(* Logix 5000 Rung export; software revision 33.00 *)

TYPE Banner_IOL_Device_SubIndex :
STRUCT
   Sub : DINT[34];
END_STRUCT
END_TYPE

TYPE Banner_IOL_QM30VT3_Device :
STRUCT
   Initial_Global_Read : BOOL;
   Command : SINT;
   Data : Banner_IOL_QM30VT3_Device_Index;
   Reset : BOOL;
END_STRUCT
END_TYPE

TYPE Banner_IOL_QM30VT3_Device_Index :
STRUCT
   Index : Banner_IOL_Device_SubIndex[19];
   Metric_Config : Banner_IOL_QM30VT3_Metric_Config;
END_STRUCT
END_TYPE

TYPE Banner_IOL_QM30VT3_Metric_Config :
STRUCT
   Metric_1 : Banner_IOL_QM30VT3_Metric_Data;
   Metric_2 : Banner_IOL_QM30VT3_Metric_Data;
   Metric_3 : Banner_IOL_QM30VT3_Metric_Data;
   Metric_4 : Banner_IOL_QM30VT3_Metric_Data;
   Metric_5 : Banner_IOL_QM30VT3_Metric_Data;
   Metric_6 : Banner_IOL_QM30VT3_Metric_Data;
   Metric_7 : Banner_IOL_QM30VT3_Metric_Data;
   Num_of_Threshold_Samples : DINT;
END_STRUCT
END_TYPE

TYPE Banner_IOL_QM30VT3_Metric_Data :
STRUCT
   Metric : DINT;   // See IODD file for all options.
   Warning_Threshold : REAL;
   Alarm_Treshold : REAL;
END_STRUCT
END_TYPE

TYPE Banner_IOL_Rules :
STRUCT
   Byte_Pos : SINT;   // Byte Position to read from or write data to.
   Multi : SINT;   // Determines if a multiple byte length index is being accessed. Use 2 for 2 bytes length, 3 for 3 byte length, etc..
   Sub_Index : SINT;
   Signed : SINT;   // 0=Unsigned, 1=Signed
END_STRUCT
END_TYPE

TYPE Banner_IOL_Rules_Array :
STRUCT
   Length : DINT;
   Settings : Banner_IOL_Rules_SettingsArray[32];
END_STRUCT
END_TYPE

TYPE Banner_IOL_Rules_SettingsArray :
STRUCT
   Index : DINT;
   Num_Op : INT;   // Number of Operations to read/write Index.
   Total_Bytes : INT;
   RW : SINT;   // 0 = Read Only, 1 = Write Only, 2 = Read or Write
   Rules : Banner_IOL_Rules[34];   // Sub Index Position in IODD.
END_STRUCT
END_TYPE

VAR_GLOBAL   (* controller tags *)
   QM30VT3_IOLM1_01 : Banner_IOL_QM30VT3_Device;
        .DATA.INDEX[2]   // Direct Parameters 1 (ro)
        .DATA.INDEX[2].SUB[1]   // Reserved
        .DATA.INDEX[2].SUB[2]   // Master Cycle Time
        .DATA.INDEX[2].SUB[3]   // Min Cycle Time
        .DATA.INDEX[2].SUB[4]   // M Sequence Capability
        .DATA.INDEX[2].SUB[5]   // IO-Link Version ID
        .DATA.INDEX[2].SUB[6]   // Process Data Input Length
        .DATA.INDEX[2].SUB[7]   // Process Data Output Length
        .DATA.INDEX[2].SUB[8]   // Vendor ID
        .DATA.INDEX[2].SUB[9]   // Device ID
        .DATA.INDEX[3]   // Standard Command (wo)
        .DATA.INDEX[3].SUB[1]   // Standard Command: 126=Locator Start, 127=Locator Stop, 129=Application Reset, 164=Reset All Metrics
        .DATA.INDEX[4]   // Serial Number (ro)
        .DATA.INDEX[4].SUB[1]   // SN1
        .DATA.INDEX[4].SUB[2]   // SN2
        .DATA.INDEX[4].SUB[3]   // SN3
        .DATA.INDEX[4].SUB[4]   // SN4
        .DATA.INDEX[4].SUB[5]   // SN5
        .DATA.INDEX[4].SUB[6]   // SN6
        .DATA.INDEX[4].SUB[7]   // SN7
        .DATA.INDEX[4].SUB[8]   // SN8
        .DATA.INDEX[4].SUB[9]   // SN9
        .DATA.INDEX[4].SUB[10]   // SN10
        .DATA.INDEX[4].SUB[11]   // SN11
        .DATA.INDEX[4].SUB[12]   // SN12
        .DATA.INDEX[4].SUB[13]   // SN13
        .DATA.INDEX[4].SUB[14]   // SN14
        .DATA.INDEX[4].SUB[15]   // SN15
        .DATA.INDEX[4].SUB[16]   // SN16
        .DATA.INDEX[5]   // All Time Run Time (ro)
        .DATA.INDEX[5].SUB[1]   // All Time Run Time
        .DATA.INDEX[6]   // Resettable Run Time
        .DATA.INDEX[6].SUB[1]   // Resettable Run Time
        .DATA.INDEX[7]   // Process Data Mode
        .DATA.INDEX[7].SUB[1]   // Process Data Mode: 0=FP Imperial, 1=SSP Imperial, 2=FP Metric, 3=SSP Metric, 4=FP User Define, 5=SSP User Define
        .DATA.INDEX[8]   // Output Configuration
        .DATA.INDEX[8].SUB[1]   // Wire Mode: 0=BannerBus, 1=Discrete Output
        .DATA.INDEX[9]   // Reserved
        .DATA.INDEX[9].SUB[1]   // Metric 1
        .DATA.INDEX[9].SUB[2]   // Metric 1 Warning Threshold
        .DATA.INDEX[9].SUB[3]   // Metric 1 Alarm Threshold
        .DATA.INDEX[9].SUB[4]   // Metric 2
        .DATA.INDEX[9].SUB[5]   // Metric 2 Warning Threshold
        .DATA.INDEX[9].SUB[6]   // Metric 2 Alarm Threshold
        .DATA.INDEX[9].SUB[7]   // Metric 3
        .DATA.INDEX[9].SUB[8]   // Metric 3 Warning Threshold
        .DATA.INDEX[9].SUB[9]   // Metric 3 Alarm Threshold
        .DATA.INDEX[9].SUB[10]   // Metric 4
        .DATA.INDEX[9].SUB[11]   // Metric 4 Warning Threshold
        .DATA.INDEX[9].SUB[12]   // Metric Alarm Threshold
        .DATA.INDEX[9].SUB[13]   // Metric 5
        .DATA.INDEX[9].SUB[14]   // Metric 5 Warning Threshold
        .DATA.INDEX[9].SUB[15]   // Metric 5 Alarm Threshold
        .DATA.INDEX[9].SUB[16]   // Metric 6
        .DATA.INDEX[9].SUB[17]   // Metric 6 Warning Threshold
        .DATA.INDEX[9].SUB[18]   // Metric 6 Alarm Threshold
        .DATA.INDEX[9].SUB[19]   // Metric 7 Alarm Threshold
        .DATA.INDEX[9].SUB[20]   // Metric 7 Warning Threshold
        .DATA.INDEX[9].SUB[21]   // Metric 7 Alarm Threshold
        .DATA.INDEX[9].SUB[22]   // Number of Threshold Samples
        .DATA.INDEX[10]   // Status (ro)
        .DATA.INDEX[10].SUB[1]   // Vibe IQ Status: 0=IDLE, 1=Start, 2=Samples Acquiring, 3=Processing, 4=Active
        .DATA.INDEX[10].SUB[2]   // Baseline Sample Left
        .DATA.INDEX[11]   // Vibe IQ Sampling
        .DATA.INDEX[11].SUB[1]   // FMAx Settings: 1=Fmax 5300 Hz, 2=Fmax 2650 Hz, 3=Fmax 1300 Hz, 4=Fmax 650 Hz, 5=Fmax 325 Hz
        .DATA.INDEX[12]   // Baseline Configuration
        .DATA.INDEX[12].SUB[1]   // Start Baseline: 0=Idle, 1=Trigger Baseline, 2=Baseline Abord/Reset
        .DATA.INDEX[12].SUB[2]   // Velocity Threshold Compare: 0=Velocity Threshold or with Axis, 1=Velocity Threshold and with Axis
        .DATA.INDEX[12].SUB[3]   // Accel Component for Threshold: 0 to 65535
        .DATA.INDEX[12].SUB[4]   // Accel Velocity or and Threshold Exceed for Baseline: 0 to 65535
        .DATA.INDEX[12].SUB[5]   // Number of Samples for Baseline: 0 to 65535
        .DATA.INDEX[12].SUB[6]   // Sample Rate in seconds for Baseline: 0 to 65535
        .DATA.INDEX[12].SUB[7]   // Number of Samples for Acute: 0 to 65535
        .DATA.INDEX[12].SUB[8]   // Number of Samples for Chronic: 0 to 65535
        .DATA.INDEX[12].SUB[9]   // Imperial or Metric Selection: 0=Imperial, 1=Metric
        .DATA.INDEX[13]   // Baseline Threshold Configuration
        .DATA.INDEX[13].SUB[1]   // X RMS Velocity Threshold for Baseline: 0 to 65535
        .DATA.INDEX[13].SUB[2]   // Y RMS Velocity Threshold for Baseline: 0 to 65535
        .DATA.INDEX[13].SUB[3]   // Z RMS Velocity Threshold for Baseline: 0 to 65535
        .DATA.INDEX[13].SUB[4]   // X RMS HP Accel Threshold for Baseline: 0 to 65535
        .DATA.INDEX[13].SUB[5]   // Y RMS HP Accel Threshold for Baseline: 0 to 65535
        .DATA.INDEX[13].SUB[6]   // Z RMS HP Accel Threshold for Baseline: 0 to 65535
        .DATA.INDEX[14]   // Baseline Avg Configuration
        .DATA.INDEX[14].SUB[1]   // X RMS Velocity Vib Baseline: 0 to 65535
        .DATA.INDEX[14].SUB[2]   // Y RMS Velocity Vib Baseline: 0 to 65535
        .DATA.INDEX[14].SUB[3]   // Z RMS Velocity Vib Baseline: 0 to 65535
        .DATA.INDEX[14].SUB[4]   // X RMS HP Accel Vibration Baseline: 0 to 65535
        .DATA.INDEX[14].SUB[5]   // Y RMS HP Accel Vibration Baseline: 0 to 65535
        .DATA.INDEX[14].SUB[6]   // Z RMS HP Accel Vibration Baseline: 0 to 65535
        .DATA.INDEX[15]   // Baseline Warning Threshold Configuration
        .DATA.INDEX[15].SUB[1]   // X RMS Velocity Warning Threshold: 0 to 65535
        .DATA.INDEX[15].SUB[2]   // Y RMS Velocity Warning Threshold: 0 to 65535
        .DATA.INDEX[15].SUB[3]   // Z RMS Velocity Warning Threshold: 0 to 65535
        .DATA.INDEX[15].SUB[4]   // X RMS HP Accel Warning Threshold: 0 to 65535
        .DATA.INDEX[15].SUB[5]   // Y RMS HP Accel Warning Threshold: 0 to 65535
        .DATA.INDEX[15].SUB[6]   // Z RMS HP Accel Warning Threshold: 0 to 65535
        .DATA.INDEX[16]   // Baseline Alarm Threshold Configuration
        .DATA.INDEX[16].SUB[1]   // X RMS Velocity Alarm Threshold: 0 to 65535
        .DATA.INDEX[16].SUB[2]   // Y RMS Velocity Alarm Threshold: 0 to 65535
        .DATA.INDEX[16].SUB[3]   // Z RMS Velocity Alarm Threshold: 0 to 65535
        .DATA.INDEX[16].SUB[4]   // X RMS HP Accel Alarm Threshold: 0 to 65535
        .DATA.INDEX[16].SUB[5]   // Y RMS HP Accel Alarm Threshold: 0 to 65535
        .DATA.INDEX[16].SUB[6]   // Z RMS HP Accel Alarm Threshold: 0 to 65535
        .DATA.INDEX[17]   // Baseline Temp Alarm Warning Threshold
        .DATA.INDEX[17].SUB[1]   // Temp Warning Treshold Value: 0 to 65535
        .DATA.INDEX[17].SUB[2]   // Temp Alarm Threshold Value: 0 to 65535
        .DATA.METRIC_CONFIG   // Index 9
   QM30VT3_Rules : Banner_IOL_Rules_Array;
        .SETTINGS[2]   // Direct Parameters 1
        .SETTINGS[2].RULES[0]   // Reserved
        .SETTINGS[2].RULES[1]   // Master Cycle Time
        .SETTINGS[2].RULES[2]   // Min Cycle Time
        .SETTINGS[2].RULES[3]   // M-Sequence Capability
        .SETTINGS[2].RULES[4]   // IO-Link ID
        .SETTINGS[2].RULES[5]   // Process Data Input Length
        .SETTINGS[2].RULES[6]   // Process Data Output Length
        .SETTINGS[2].RULES[7]   // Vendor ID
        .SETTINGS[2].RULES[8]   // Device ID
        .SETTINGS[3]   // Standard Command
        .SETTINGS[3].RULES[0]   // Standard Command
        .SETTINGS[4]   // Serial Number
        .SETTINGS[4].RULES[0]   // SN1
        .SETTINGS[4].RULES[1]   // SN2
        .SETTINGS[4].RULES[2]   // SN3
        .SETTINGS[4].RULES[3]   // SN4
        .SETTINGS[4].RULES[4]   // SN5
        .SETTINGS[4].RULES[5]   // SN6
        .SETTINGS[4].RULES[6]   // SN7
        .SETTINGS[4].RULES[7]   // SN8
        .SETTINGS[4].RULES[8]   // SN9
        .SETTINGS[4].RULES[9]   // SN10
        .SETTINGS[4].RULES[10]   // SN11
        .SETTINGS[4].RULES[11]   // SN12
        .SETTINGS[4].RULES[12]   // SN13
        .SETTINGS[4].RULES[13]   // SN14
        .SETTINGS[4].RULES[14]   // SN15
        .SETTINGS[4].RULES[15]   // SN16
        .SETTINGS[5]   // All Time Run Time
        .SETTINGS[5].RULES[0]   // All Time Run Time
        .SETTINGS[6]   // Resettable Run Time
        .SETTINGS[6].RULES[0]   // Resettable Run Time
        .SETTINGS[7]   // Process Data Mode
        .SETTINGS[7].RULES[0]   // Process Data Mode
        .SETTINGS[8]   // Output Configuration
        .SETTINGS[8].RULES[0]   // Output Configuration
        .SETTINGS[9]   // Metric Configuration
        .SETTINGS[9].RULES[0]   // Metric 1
        .SETTINGS[9].RULES[1]   // Metric 1 Warning Threshold
        .SETTINGS[9].RULES[2]   // Metric 1 Alarm Threshold
        .SETTINGS[9].RULES[3]   // Metric 2
        .SETTINGS[9].RULES[4]   // Metric 2 Warning Threshold
        .SETTINGS[9].RULES[5]   // Metric 2 Alarm Threshold
        .SETTINGS[9].RULES[6]   // Metric 3
        .SETTINGS[9].RULES[7]   // Metric 3 Warning Threshold
        .SETTINGS[9].RULES[8]   // Metric 3 Alarm Threshold
        .SETTINGS[9].RULES[9]   // Metric 4
        .SETTINGS[9].RULES[10]   // Metric 4 Warning Threshold
        .SETTINGS[9].RULES[11]   // Metric 4 Alarm Threshold
        .SETTINGS[9].RULES[12]   // Metric 5
        .SETTINGS[9].RULES[13]   // Metric 5 Warning Threshold
        .SETTINGS[9].RULES[14]   // Metric 5 Alarm Threshold
        .SETTINGS[9].RULES[15]   // Metric 6
        .SETTINGS[9].RULES[16]   // Metric 6 Warning Threshold
        .SETTINGS[9].RULES[17]   // Metric 6 Alarm Threshold
        .SETTINGS[9].RULES[18]   // Metric 7
        .SETTINGS[9].RULES[19]   // Metric 7 Warning Threshold
        .SETTINGS[9].RULES[20]   // Metric 7 Alarm Threshold
        .SETTINGS[9].RULES[21]   // Number of Threshold Samples
        .SETTINGS[10]   // Status
        .SETTINGS[10].RULES[0]   // Vibe IQ Status
        .SETTINGS[10].RULES[1]   // Baseline Sample Left
        .SETTINGS[11]   // Vibe IQ Sampling
        .SETTINGS[11].RULES[0]   // FMax Settings
        .SETTINGS[12]   // Baseline Configuration
        .SETTINGS[12].RULES[0]   // Start Baseline
        .SETTINGS[12].RULES[1]   // Velocity Threshold Compare
        .SETTINGS[12].RULES[2]   // Accel Component for Threshold
        .SETTINGS[12].RULES[3]   // Accel Velocity or and Threshold Exceed for Baseline
        .SETTINGS[12].RULES[4]   // Number of Samples for Baseline
        .SETTINGS[12].RULES[5]   // Sample Rate in seconds for Baseline
        .SETTINGS[12].RULES[6]   // Number of Samples for Acute
        .SETTINGS[12].RULES[7]   // Number of Samples for Chronic
        .SETTINGS[12].RULES[8]   // Imperial or Metric Selection
        .SETTINGS[13]   // Baseline Threshold Configuration
        .SETTINGS[13].RULES[0]   // X RMS Velocity Threshold for Baseline
        .SETTINGS[13].RULES[1]   // Y RMS Velocity Threshold for Baseline
        .SETTINGS[13].RULES[2]   // Z RMS Velocity Threshold for Baseline
        .SETTINGS[13].RULES[3]   // X RMS HP Accel Threshold for Baseline
        .SETTINGS[13].RULES[4]   // Y RMS HP Accel Threshold for Baseline
        .SETTINGS[13].RULES[5]   // Z RMS HP Accel Threshold for Baseline
        .SETTINGS[14]   // Baseline Avg Configuration
        .SETTINGS[14].RULES[0]   // X RMS Velocity Baseline Value
        .SETTINGS[14].RULES[1]   // Y RMS Velocity Baseline Value
        .SETTINGS[14].RULES[2]   // Z RMS Velocity Baseline Value
        .SETTINGS[14].RULES[3]   // X RMS HP Accel Baseline Value
        .SETTINGS[14].RULES[4]   // Y RMS HP Accel Baseline Value
        .SETTINGS[14].RULES[5]   // Z RMS HP Accel Baseline Value
        .SETTINGS[15]   // Baseline Warning Threhsold Configuration
        .SETTINGS[15].RULES[0]   // X RMS Velocity Warning Threshold
        .SETTINGS[15].RULES[1]   // Y RMS Velocity Warning Threshold
        .SETTINGS[15].RULES[2]   // Z RMS Velocity Warning Threshold
        .SETTINGS[15].RULES[3]   // X RMS HP Accel Warning Threshold
        .SETTINGS[15].RULES[4]   // Y RMS HP Accel Warning Threshold
        .SETTINGS[15].RULES[5]   // Z RMS HP Accel Warning Threshold
        .SETTINGS[16]   // Baseline Alarm Threshold Configuration
        .SETTINGS[16].RULES[0]   // X RMS Velocity Alarm Threshold
        .SETTINGS[16].RULES[1]   // Y RMS Velocity Alarm Threshold
        .SETTINGS[16].RULES[2]   // Z RMS Velocity Alarm Threshold
        .SETTINGS[16].RULES[3]   // X RMS HP Accel Alarm Threshold
        .SETTINGS[16].RULES[4]   // Y RMS HP Accel Alarm Threshold
        .SETTINGS[16].RULES[5]   // Z RMS HP Accel Alarm Threshold
        .SETTINGS[17]   // Baseline Temp Alarm Warning Threshold
        .SETTINGS[17].RULES[0]   // Temp Warning Threshold Value
        .SETTINGS[17].RULES[1]   // Temp Alarm Threshold Value
END_VAR

PROGRAM MainProgram

ROUTINE MainRoutine   (* ladder *)
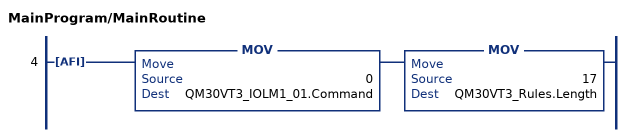
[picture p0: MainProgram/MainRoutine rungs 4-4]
   4: AFI()MOV(0,QM30VT3_IOLM1_01.Command)MOV(17,QM30VT3_Rules.Length);
END_ROUTINE
END_PROGRAM
